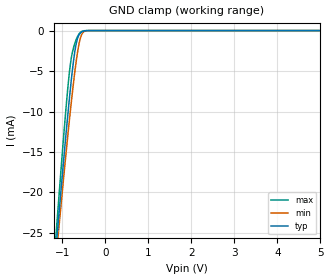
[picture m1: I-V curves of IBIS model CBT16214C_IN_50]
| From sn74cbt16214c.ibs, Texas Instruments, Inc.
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[Model]   CBT16214C_IN_50
Model_type  Input
Vinl=0.8
Vinh=2.0
| variable   typ   min   max
C_comp   2.13pF   1.47pF   2.96pF
[Temperature Range]   40   100   -40
| Ambient temperature   25   85   -40
[Voltage range]   5   4.5   5.5
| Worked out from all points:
|   GND clamp passes 1 mA (typ) near -0.64 V on its own axis
[GND Clamp]
| CBT16214C_IN_50
|   Voltage   I(typ)   I(min)   I(max)
-5V       -302.1mA   -280.3mA   -328.8mA
-1.16V    -28.09mA   -29.24mA   -26.56mA
-1.125V   -25.87mA   -27.21mA   -24.06mA
-1.09V    -23.67mA   -25.19mA   -21.6mA
-1.06V    -21.8mA    -23.48mA   -19.51mA
-910mV    -12.78mA   -15.18mA   -9.584mA
-815mV    -7.535mA   -10.23mA   -4.436mA
-760mV    -4.828mA   -7.553mA   -2.642mA
-680mV    -1.806mA   -4.061mA   -1.212mA
-605mV    -517.2uA   -1.574mA   -394.6uA
-545mV    -167.7uA   -480.6uA   -102.3uA
5V        123.2pA    299.2pA    65.41pA
